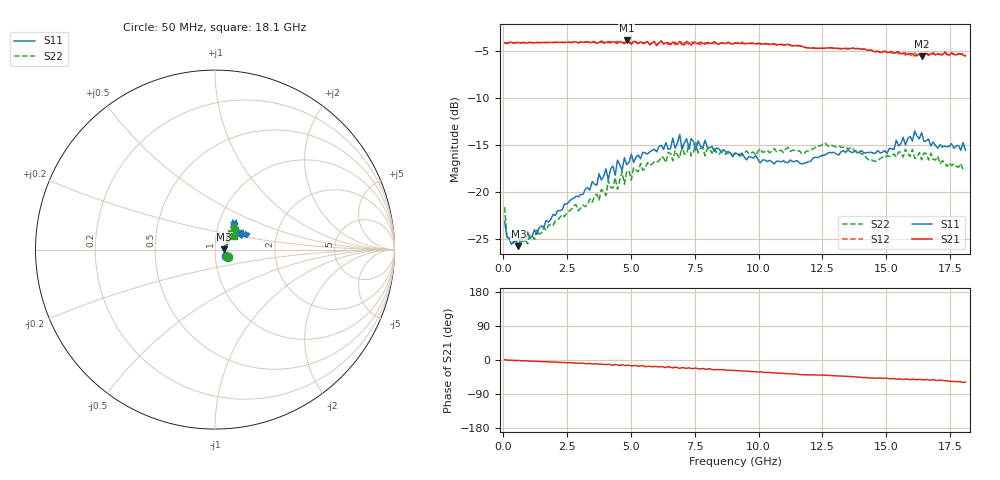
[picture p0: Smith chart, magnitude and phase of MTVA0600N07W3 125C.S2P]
! Network Analyzer HP8720D.06.14 Serial No. US36140669
!  8 Jul 2005  12:47:02
! Frequency  S11  S21  S12  S22
# HZ  S  DB R 50
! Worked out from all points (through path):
!   201 points, 50 MHz to 18.1 GHz, reference 50 ohm
!   highest |S21| = -3.82 dB at 4.833 GHz (marker M1); lowest = -5.5 dB at 16.39 GHz (marker M2)
!   group delay of S21, straight-line fit = 9.14 ps
!   lowest |S11| = -25.8 dB at 591.5 MHz (marker M3), VSWR 1.11, Z = 55.4 + j0.27 ohm
!   |S11| at or under -10 dB: start of sweep to end of sweep
!   |S22| runs from -25.6 to -14.8 dB; largest |S21 - S12| = 0.031
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5e7  -23.13 -31.9  -4.06 0.7  -4.08 0.9  -21.63 -29.4
1.4025e8  -24.83 -17.6  -4.16 0.0  -4.15 -0.1  -24.69 -15.8
5.915e8  -25.80 2.7  -4.04 -1.1  -4.11 -1.3  -24.90 5.2
9.525e8  -24.31 10.5  -4.10 -2.6  -4.02 -2.7  -25.56 10.8
3.1185e9  -20.27 35.2  -4.00 -8.2  -4.05 -8.6  -21.39 39.7
4.021e9  -17.53 41.7  -4.04 -12.3  -3.99 -11.3  -20.42 43.7
4.11125e9  -18.73 42.2  -3.93 -11.1  -4.08 -12.2  -18.77 44.7
4.382e9  -18.22 42.7  -4.00 -11.9  -4.07 -13.3  -18.45 47.5
4.47225e9  -16.60 40.1  -4.14 -13.0  -3.91 -12.6  -19.72 51.1
4.83325e9  -17.10 49.8  -3.82 -14.5  -4.07 -14.6  -17.83 43.2
6.09675e9  -15.15 48.8  -4.10 -18.6  -3.98 -18.5  -16.72 49.7
6.7285e9  -15.34 56.1  -4.02 -18.4  -4.29 -18.9  -15.60 47.0
6.909e9  -13.86 54.1  -3.93 -21.9  -3.96 -20.2  -16.38 47.3
6.99925e9  -15.49 54.1  -4.10 -20.0  -4.31 -21.7  -14.99 48.8
7.36025e9  -14.32 50.1  -4.32 -22.3  -3.99 -21.9  -16.16 52.6
7.54075e9  -15.52 52.2  -4.05 -21.1  -4.00 -23.9  -14.76 51.2
7.90175e9  -14.49 55.1  -4.22 -24.4  -4.06 -23.1  -16.16 47.3
9.075e9  -15.84 53.5  -4.10 -27.9  -4.07 -28.0  -15.93 41.3
1.21435e10  -16.36 39.4  -4.64 -39.3  -4.58 -39.5  -15.40 43.9
1.512175e10  -15.35 26.1  -5.11 -49.5  -4.93 -49.2  -16.21 42.9
1.638525e10  -13.68 23.9  -5.53 -51.6  -5.26 -51.1  -16.59 39.6
1.81e10  -15.54 32.8  -5.44 -58.2  -5.58 -58.7  -17.60 35.6
